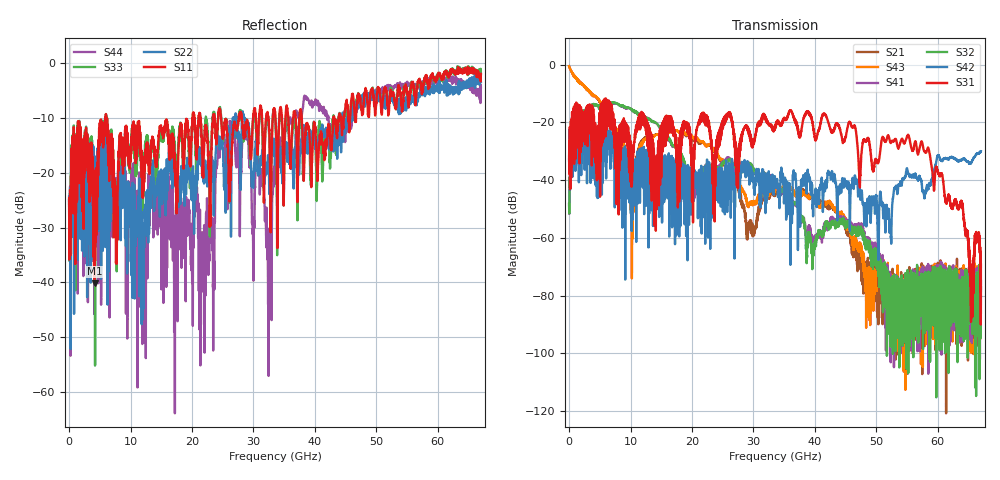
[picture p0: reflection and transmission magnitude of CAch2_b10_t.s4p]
!Agilent Technologies,N5247A,US51170199,A.09.90.13
!Agilent N5247A: A.09.90.13
!Date: Tuesday, October 23, 2018 14:01:20
!Correction: S11(Full 4 Port(1,2,3,4))
!S12(Full 4 Port(1,2,3,4))
!S13(Full 4 Port(1,2,3,4))
!S14(Full 4 Port(1,2,3,4))
!S21(Full 4 Port(1,2,3,4))
!S22(Full 4 Port(1,2,3,4))
!S23(Full 4 Port(1,2,3,4))
!S24(Full 4 Port(1,2,3,4))
!S31(Full 4 Port(1,2,3,4))
!S32(Full 4 Port(1,2,3,4))
!S33(Full 4 Port(1,2,3,4))
!S34(Full 4 Port(1,2,3,4))
!S41(Full 4 Port(1,2,3,4))
!S42(Full 4 Port(1,2,3,4))
!S43(Full 4 Port(1,2,3,4))
!S44(Full 4 Port(1,2,3,4))
!S4P File: Measurements: <S11,S12,S13,S14>,
!<S21,S22,S23,S24>,
!<S31,S32,S33,S34>,
!<S41,S42,S43,S44>:
# Hz S  dB  R 50
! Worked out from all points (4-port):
!   6701 points, 10 MHz to 67 GHz, reference 50 ohm
!   strongest paths, dB at 10 MHz, 16.76 GHz, 33.51 GHz, 50.25 GHz, 67 GHz:
!     S31: -32.8, -23.2, -21.1, -34.1, -69.2
!     S42: -33.3, -46.6, -39.8, -57.4, -30.1
!     S32: -48.3, -27.5, -41.9, -69.9, -77.1
!     S41: -48.3, -27.7, -41.9, -66.0, -74.8
!     S43: -0.6, -22.8, -43.8, -69.5, -85.8
!     S21: -0.6, -22.9, -45.1, -81.8, -82.8
!   lowest |S11| = -40.1 dB at 4.149 GHz (marker M1), VSWR 1.02, Z = 49.3 - j0.701 ohm
!   |S11| at or under -10 dB: start of sweep to 5.878 GHz; 6.1 GHz to 20.13 GHz (14.03 GHz wide, 107 % of centre); 37.86 GHz to 42.98 GHz (5.122 GHz wide, 12.7 % of centre)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
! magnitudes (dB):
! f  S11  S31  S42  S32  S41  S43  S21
! 10 MHz  -25.0  -32.8  -33.3  -48.3  -48.3  -0.6  -0.6
! 4.149 GHz  -40.1  -23.1  -28.2  -13.9  -13.9  -10.8  -10.8
! 10.23 GHz  -12.4  -41.4  -38.2  -15.8  -15.8  -70.2  -38.2
! 12.01 GHz  -22.1  -19.4  -33.6  -17.7  -17.6  -26.4  -25.9
! 18.68 GHz  -16.0  -20.3  -39.7  -33.5  -34.9  -23.6  -23.9
! 55.13 GHz  -6.9  -24.4  -37.4  -84.3  -74.2  -83.4  -89.4
! 67 GHz  -2.0  -69.2  -30.1  -77.1  -74.8  -85.8  -82.8
